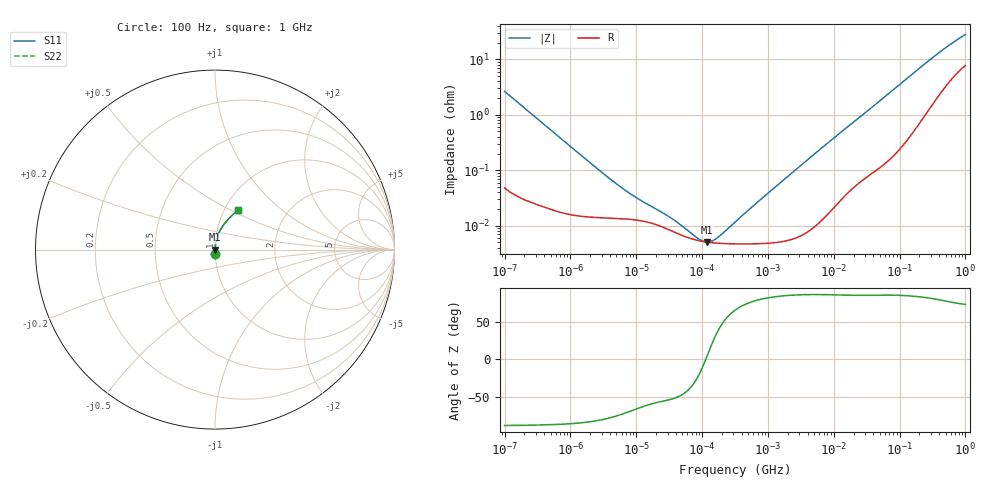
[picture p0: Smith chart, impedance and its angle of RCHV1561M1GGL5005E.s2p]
! RCHV1561M1GGL5005E  S-PARAMETER MODEL  (AEC-Q200 qualified)
! Model Generated by ELNA Corporation (http://www.ty-top.com)
! Version 1.0
! ELNA Control No. 240229
! Copyright (c) 2024 ELNA CO.,LTD. All Rights Reserved.
! Products Name : CONDUCTIVE POLYMER HYBRID ALUMINUM ELECTROLYTIC CAPACITORS
! Characteristics :
!  Capacitance  :  560uF  ,  Rated voltage  :  35V
!  Operating Temp. Range  :  -55 to +105 degC  ,  Endurance  :  10000hr at 105 degC
!  Dimension D  :  12.5mm  ,  Dimension L  :  13.5mm
! Frequency Range : 100Hz - 1GHz
! External Node Assignments :
!  1  o---| |---o  2
# MHz S RI R 50
!Freq[MHz].  S11 Real  S11 Imag  S21 Real  S21 Imag  S12 Real  S12 Imag  S22 Real  S22 Imag
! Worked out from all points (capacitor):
!   401 points, 100 Hz to 1 GHz, reference 50 ohm
!   read as one part in series: C = 601 uF near 108 Hz
!   lowest |Z| = 5.09 mohm at 120.2 kHz (marker M1)
!   series resonance near 113.7 kHz, so ESL is about 3.3 nH
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0.0001  0.00118 -0.0264  0.9988 0.0264  0.9988 0.0264  0.00118 -0.0264
0.000113  0.000979 -0.0234  0.999 0.0234  0.999 0.0234  0.000979 -0.0234
0.001488  0.000151 -0.00181  0.9998 0.00181  0.9998 0.00181  0.000151 -0.00181
0.003758  0.000138 -0.000727  0.9999 0.000727  0.9999 0.000727  0.000138 -0.000727
0.006607  0.000133 -0.000426  0.9999 0.000426  0.9999 0.000426  0.000133 -0.000426
0.011156  0.000124 -0.00027  0.9999 0.00027  0.9999 0.00027  0.000124 -0.00027
0.022131  0.000101 -0.000158  0.9999 0.000158  0.9999 0.000158  0.000101 -0.000158
0.049545  6.7e-05 -7.34e-05  0.9999 7.34e-05  0.9999 7.34e-05  6.7e-05 -7.34e-05
0.053703  6.45e-05 -6.58e-05  0.9999 6.58e-05  0.9999 6.58e-05  6.45e-05 -6.58e-05
0.120226  5.06e-05 4.82e-06  0.9999 -4.82e-06  0.9999 -4.82e-06  5.06e-05 4.82e-06
0.258523  4.74e-05 8.04e-05  1 -8.04e-05  1 -8.04e-05  4.74e-05 8.04e-05
0.280221  4.73e-05 9.04e-05  1 -9.04e-05  1 -9.04e-05  4.73e-05 9.04e-05
0.316228  4.72e-05 0.000106  1 -0.000106  1 -0.000106  4.72e-05 0.000106
0.798914  4.78e-05 0.000303  1 -0.000303  1 -0.000303  4.78e-05 0.000303
4.704354  9.17e-05 0.00181  0.9999 -0.00181  0.9999 -0.00181  9.17e-05 0.00181
24.54709  0.000677 0.00896  0.9993 -0.00896  0.9993 -0.00896  0.000677 0.00896
69.9842  0.00214 0.0246  0.9979 -0.0246  0.9979 -0.0246  0.00214 0.0246
169.8244  0.00866 0.0579  0.9913 -0.0579  0.9913 -0.0579  0.00866 0.0579
365.1741  0.0327 0.1145  0.9673 -0.1145  0.9673 -0.1145  0.0327 0.1145
641.9482  0.076 0.1713  0.924 -0.1713  0.924 -0.1713  0.076 0.1713
922.5714  0.1164 0.2099  0.8836 -0.2099  0.8836 -0.2099  0.1164 0.2099
1000  0.1264 0.2188  0.8736 -0.2188  0.8736 -0.2188  0.1264 0.2188
